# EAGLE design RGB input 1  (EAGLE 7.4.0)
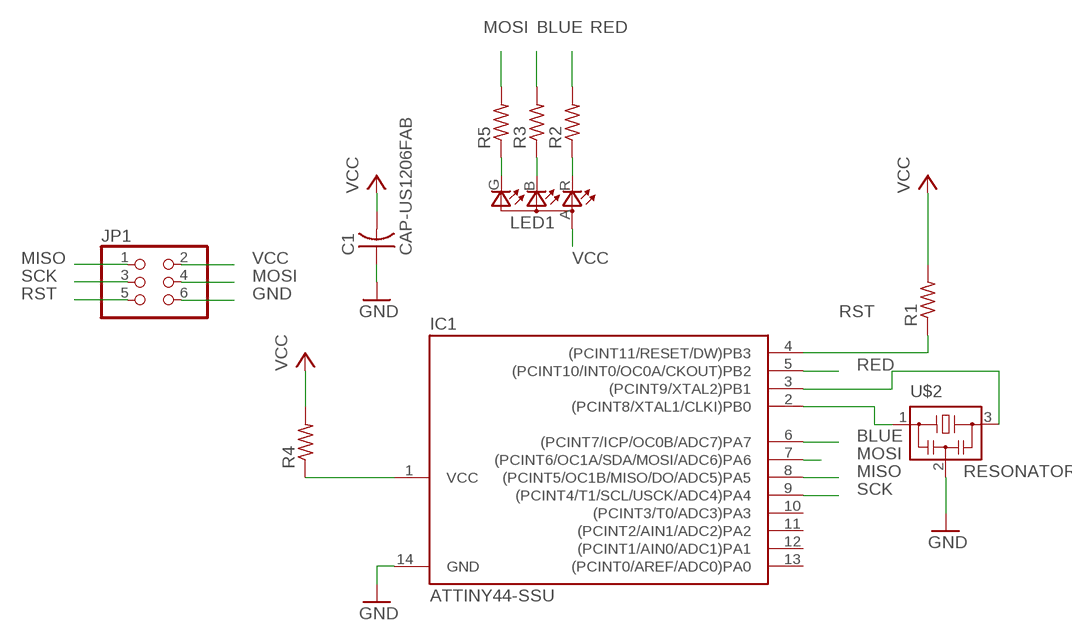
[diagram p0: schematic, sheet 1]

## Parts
C1  CAP-US1206FAB  [C1206FAB]
IC1  ATTINY44-SSU  [SOIC14]
JP1  PINHD-2X3-SMD  [2X03SMD]
LED1  LEDRGBOLD  [P-LCC-4-3]
R1  RES-US1206FAB  [R1206FAB]
R2  RES-US1206FAB  [R1206FAB]
R3  RES-US1206FAB  [R1206FAB]
R4  RES-US1206FAB  [R1206FAB]
R5  RES-US1206FAB  [R1206FAB]
U$2  RESONATOR  [EFOBM]

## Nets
BLUE: IC1.6((PCINT7/ICP/OC0B/ADC7)PA7) R3.2
GND: C1.1 IC1.14(GND) JP1.6 U$2.2
MISO: IC1.8((PCINT5/OC1B/MISO/DO/ADC5)PA5) JP1.1
MOSI: IC1.7((PCINT6/OC1A/SDA/MOSI/ADC6)PA6) JP1.4 R5.2
N$1: LED1.B(CBLUE) R3.1
N$2: IC1.3((PCINT9/XTAL2)PB1) U$2.3
N$3: IC1.2((PCINT8/XTAL1/CLKI)PB0) U$2.1
N$4: LED1.R(CRED) R2.1
N$5: IC1.1(VCC) R4.1
N$6: LED1.G(CGREEN) R5.1
RED: IC1.5((PCINT10/INT0/OC0A/CKOUT)PB2) R2.2
RST: IC1.4((PCINT11/RESET/DW)PB3) JP1.5 R1.1
SCK: IC1.9((PCINT4/T1/SCL/USCK/ADC4)PA4) JP1.3
VCC: C1.2 JP1.2 LED1.A(A2) R1.2 R4.2
Unconnected: IC1.10((PCINT3/T0/ADC3)PA3) IC1.11((PCINT2/AIN1/ADC2)PA2) IC1.12((PCINT1/AIN0/ADC1)PA1) IC1.13((PCINT0/AREF/ADC0)PA0)

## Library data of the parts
C1 = fab:CAP-US
IC1 = fab:ATTINY44
JP1 = fab:PINHD-2X3-SMD: PIN HEADER
LED1 = fab:LEDRGBOLD: OSRAM Hyper Multi TOPLED® Hyper-Bright LED LATB T686 Source: http://www.osram.convergy.de/
R1-R5 = fab:RES-US: Resistor (US Symbol)
U$2 = fab:RESONATOR

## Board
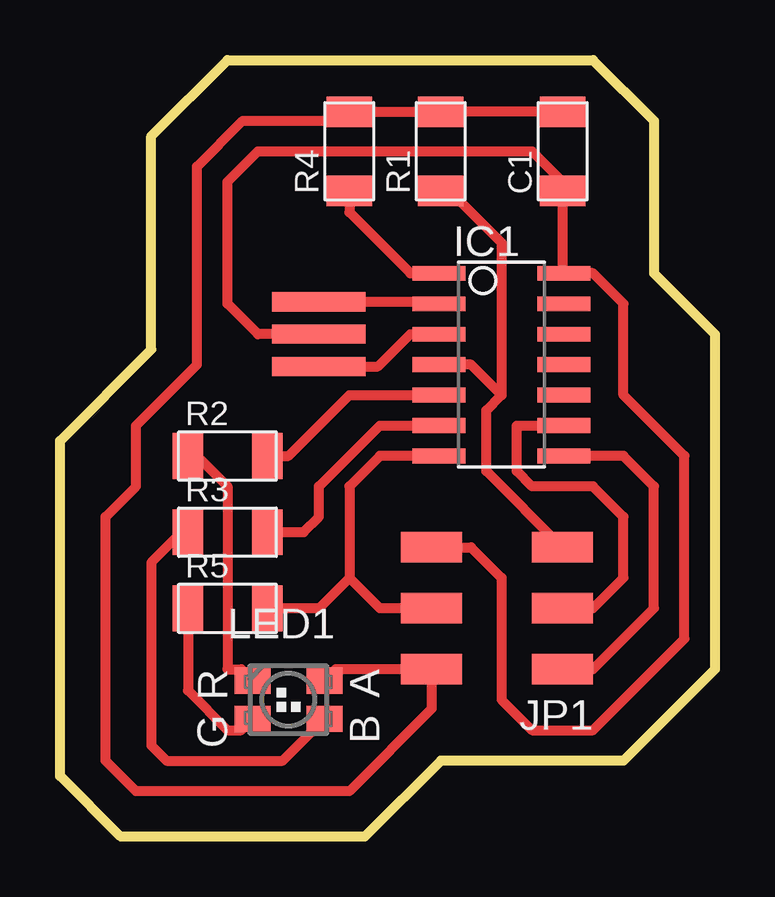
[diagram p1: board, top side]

Size 27.3 x 32.39 mm. Coordinates in mm from the lower left corner, seen from the top.
Outline: 24.77,29.84 24.77,23.5 27.3,20.96 27.3,6.99 23.49,3.18 15.88,3.18 12.7,0 2.54,0 0,2.54 0,16.51 3.81,20.32 3.81,29.21 6.98,32.39 22.23,32.39 24.77,29.84
Copper layers (1*16): Top 0.035mm / dielectric 1.5mm / Bottom 0.035mm
Design rules "default": minimum track width 10mil, minimum drill 24mil, track to track 8mil, track to pad 8mil, pad to pad 8mil, via to via 8mil, smd to smd 8mil, copper to edge 40mil, drill to drill 8mil, minimum pad ring 10mil, minimum via ring 8mil, stop-mask expansion 4mil, vias tented up to drill 0mil, thermal gap 10mil

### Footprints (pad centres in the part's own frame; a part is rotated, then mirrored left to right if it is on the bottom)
C1206FAB = smd 1.27 x 1.905: 1 -1.651,0; 2 1.651,0
SOIC14 = smd 0.61 x 2.21: 1 -3.81,-2.603; 2 -2.54,-2.603; 3 -1.27,-2.603; 4 0,-2.603; 5 1.27,-2.603; 6 2.54,-2.603; 7 3.81,-2.603; 8 3.81,2.603; 9 2.54,2.603; 10 1.27,2.603; 11 0,2.603; 12 -1.27,2.603; 13 -2.54,2.603; 14 -3.81,2.603
2X03SMD = smd 2.54 x 1.27: 1 -2.54,2.54; 2 2.92,2.54; 3 -2.54,0; 4 2.92,0; 5 -2.54,-2.54; 6 2.92,-2.54
P-LCC-4-3 = smd 1.1 x 1.5: A -0.8,1.5; B 0.8,1.5; G 0.8,-1.5; R -0.8,-1.5
R1206FAB = smd 1.27 x 1.905: 1 -1.651,0; 2 1.651,0
EFOBM = smd 0.8 x 3.9: 1 -1.35,0; 2 0,0; 3 1.35,0

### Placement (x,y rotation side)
C1  20.95,28.58 90 top
IC1  18.41,19.69 270 top
JP1  18.41,9.53 180 top
LED1  9.52,5.72 270 top
R1  15.88,28.58 90 top
R2  6.98,15.88 0 top
R3  6.98,12.7 0 top
R4  12.06,28.58 90 top
R5  6.98,9.53 0 top
U$2  10.8,20.96 270 top

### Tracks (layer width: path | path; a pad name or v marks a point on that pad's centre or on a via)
BLUE
  Top 0.406: R3.2 10.16,12.7 10.8,13.33 10.8,14.61 13.34,17.15 IC1.6
GND
  Top 0.406: U$2.2 8.25,20.96 6.98,22.23 6.98,27.3 8.25,28.58 19.68,28.58 20.95,27.3 C1.1 20.95,23.56 IC1.14 22.23,23.5 23.49,22.23 23.49,18.41 26.03,15.88 26.03,8.26 22.23,4.45 19.68,4.45 18.41,5.72 18.41,10.79 17.14,12.06 JP1.6
MISO
  Top 0.406: JP1.1 22.23,6.99 24.77,9.53 24.77,14.61 23.49,15.88 IC1.8
MOSI
  Top 0.406: IC1.7 13.34,15.88 12.06,14.61 12.06,10.79 | 12.06,10.79 10.8,9.53 R5.2 | JP1.4 13.34,9.53 12.06,10.79
N$1
  Top 0.406: R3.1 5.08,12.7 3.81,11.43 3.81,3.81 4.45,3.18 9.29,3.18 LED1.B
N$2
  Top 0.406: U$2.3 13.25,19.61 14.6,20.96 IC1.3
N$3
  Top 0.406: U$2.1 15.73,22.3 IC1.2
N$4
  Top 0.406: R2.1 5.71,15.88 6.98,14.61 6.98,6.99 7.55,6.99 LED1.R
N$5
  Top 0.406: R4.1 12.06,26.04 14.6,23.5 IC1.1
N$6
  Top 0.406: R5.1 5.33,6.1 6.98,4.45 7.55,4.45 LED1.G
RED
  Top 0.406: R2.2 9.52,15.88 12.06,18.41 IC1.5
RST
  Top 0.406: 18.41,18.41 17.14,19.69 IC1.4 | R1.1 16.26,26.92 18.41,24.77 18.41,18.41 | JP1.5 17.78,15.24 17.78,17.78 18.41,18.41
SCK
  Top 0.406: JP1.3 22.23,9.53 23.49,10.79 23.49,13.33 22.23,14.61 19.68,14.61 19.05,15.24 19.05,17.15 IC1.9
VCC
  Top 0.406: LED1.A 11.49,6.99 JP1.2 15.49,5.33 12.06,1.91 3.17,1.91 1.9,3.18 1.9,13.33 3.17,14.61 3.17,17.15 5.71,19.69 5.71,27.94 7.62,29.84 11.68,29.84 R4.2 R1.2 C1.2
